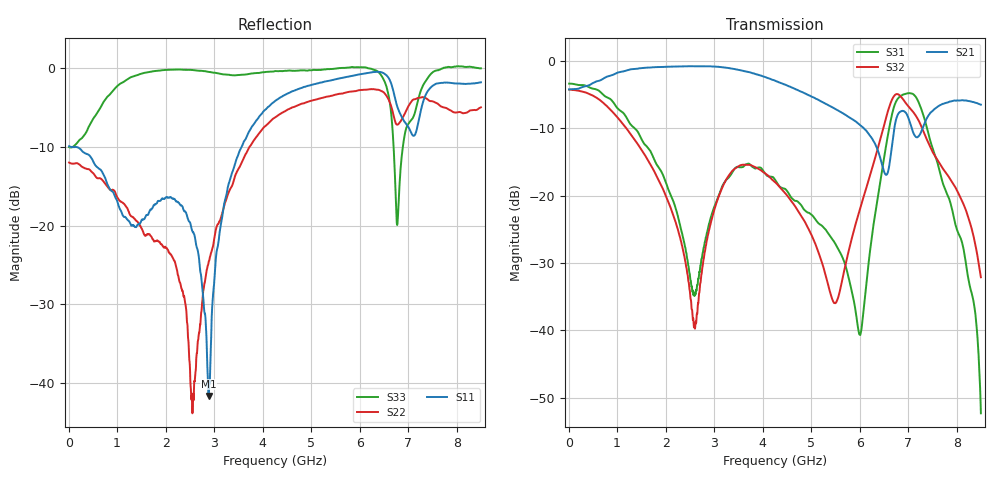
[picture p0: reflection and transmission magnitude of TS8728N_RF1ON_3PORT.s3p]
!Created with skrf (http://scikit-rf.org).
# GHz S RI R 50.0
!freq ReS11 ImS11 ReS12 ImS12 ReS13 ImS13
! ReS21 ImS21 ReS22 ImS22 ReS23 ImS23
! ReS31 ImS31 ReS32 ImS32 ReS33 ImS33
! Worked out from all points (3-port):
!   1601 points, 10 MHz to 8.5 GHz, reference 50 ohm
!   strongest paths, dB at 10 MHz, 2.132 GHz, 4.255 GHz, 6.378 GHz, 8.5 GHz:
!     S21: -4.2, -0.9, -2.9, -13.3, -6.5
!     S32: -4.3, -22.4, -18.0, -12.9, -32.1
!     S31: -3.4, -20.4, -17.6, -20.1, -52.3
!   lowest |S11| = -41.6 dB at 2.886 GHz (marker M1), VSWR 1.02, Z = 50.6 + j0.534 ohm
!   |S11| at or under -10 dB: 38.74 MHz to 3.571 GHz (3.532 GHz wide, 196 % of centre)
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0.01  -0.3189 0.00781  0.6144 0.00279  0.6777 -0.00742
      0.6142 0.00267  -0.2509 0.00795  0.6118 -0.00856
      0.6776 -0.00756  0.612 -0.00837  -0.314 0.0173
1.278194  0.07 0.0737  0.8152 -0.289  -0.036 -0.3353
          0.8152 -0.2888  -0.0259 0.1127  -0.0643 -0.2793
          -0.0361 -0.3355  -0.0643 -0.279  0.8601 -0.1459
2.551694  0.0623 -0.0676  0.4693 -0.782  -0.00115 -0.0194
          0.4693 -0.7823  0.00278 0.00581  -0.012 0.00608
          -0.0012 -0.0194  -0.0119 0.00609  0.3571 -0.9029
2.885988  0.00639 0.00527  0.3118 -0.8551  0.0575 -0.0158
          0.3117 -0.8551  0.0154 -0.0564  0.0483 0.0225
          0.0574 -0.0158  0.0486 0.0225  -0.00254 -0.9436
4.255  -0.4921 0.3711  -0.3228 -0.636  -0.0343 -0.1272
       -0.3246 -0.6351  -0.4654 0.1367  -0.0232 -0.1238
       -0.0345 -0.1269  -0.0229 -0.124  -0.6332 0.7164
5.48605  -0.6922 0.4843  -0.3841 -0.2184  -0.0321 -0.0313
         -0.3841 -0.2183  -0.0505 0.6728  0.00571 -0.0149
         -0.0321 -0.0313  0.00569 -0.0149  -0.437 0.886
6.006062  -0.788 0.4592  -0.3152 -0.1129  -0.00666 0.00648
          -0.3153 -0.1123  0.3013 0.6572  0.0795 -0.00453
          -0.00662 0.0065  0.0796 -0.00442  -0.5197 0.8643
7.130987  0.2801 0.2466  -0.2378 -0.1493  -0.3888 -0.3963
          -0.238 -0.1491  0.5578 0.2997  -0.3153 -0.2563
          -0.3884 -0.3953  -0.3145 -0.2557  -0.4083 -0.3051
7.497119  0.1739 -0.7476  -0.3146 -0.2835  -0.2048 0.1015
          -0.3138 -0.2837  0.6147 -0.00531  -0.212 -0.0254
          -0.2055 0.1011  -0.2117 -0.0253  -0.7452 -0.5606
8.5  0.0855 -0.8064  -0.4411 0.1672  0.000985 0.00218
     -0.442 0.1683  -0.4491 -0.3385  -0.0249 -0.000486
     0.001 0.00221  -0.0248 -0.000601  -0.6745 -0.7304
